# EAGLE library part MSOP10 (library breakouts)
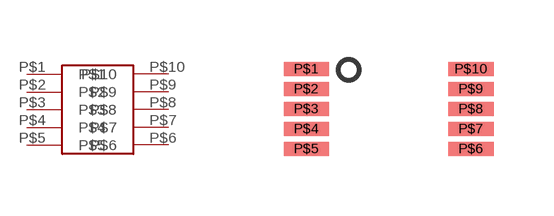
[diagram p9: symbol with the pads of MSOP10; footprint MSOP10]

Designator prefix -

## MSOP10MSOP  [MSOP10]
P$1  P$1
P$2  P$2
P$3  P$3
P$4  P$4
P$5  P$5
P$6  P$6
P$7  P$7
P$8  P$8
P$9  P$9
P$10  P$10

## Footprint MSOP10 (pad centres in mm)
smd 1.13 x 0.35: P$1 -2.06,1; P$2 -2.06,0.5; P$3 -2.06,0; P$4 -2.06,-0.5; P$5 -2.06,-1; P$6 2.06,-1; P$7 2.06,-0.5; P$8 2.06,0; P$9 2.06,0.5; P$10 2.06,1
